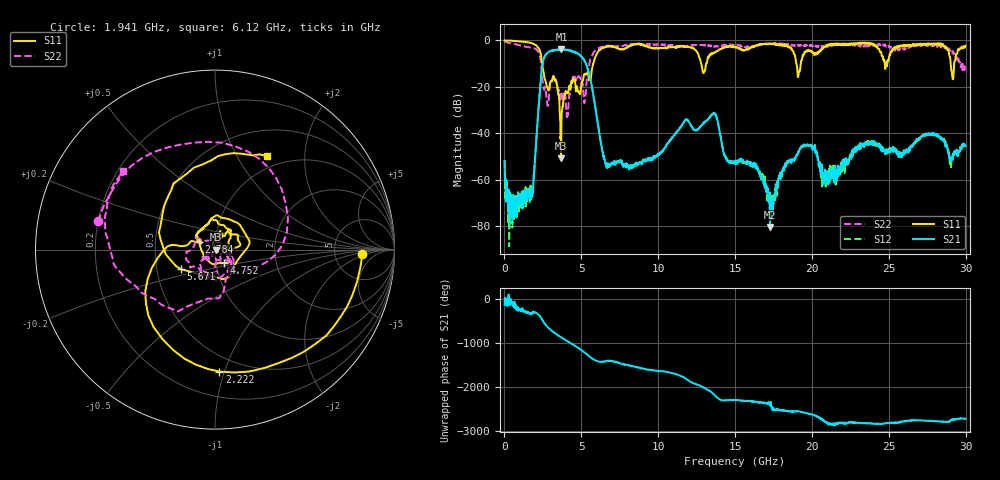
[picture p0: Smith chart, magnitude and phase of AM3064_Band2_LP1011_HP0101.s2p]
# Hz S DB R 50.0
!freq dBS11 angS11 dBS21 angS21 dBS12 angS12 dBS22 angS22
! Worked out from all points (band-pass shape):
!   1600 points, 10 MHz to 29.98 GHz, reference 50 ohm
!   highest |S21| = -3.77 dB at 3.703 GHz (marker M1); lowest = -80.2 dB at 17.27 GHz (marker M2)
!   |S21| within 3 dB of the highest: 2.628 GHz to 4.979 GHz (2.351 GHz wide, 61.8 % of centre)
!   lowest |S11| = -50.7 dB at 3.684 GHz (marker M3), VSWR 1.01, Z = 50.3 + j0.055 ohm
!   |S11| at or under -10 dB: 2.45 GHz to 5.773 GHz (3.323 GHz wide, 80.8 % of centre); 12.8 GHz to 13.12 GHz (321.1 MHz wide, 2.48 % of centre); 18.98 GHz to 19.27 GHz (290.4 MHz wide, 1.52 % of centre)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
!   |S22| runs from -33.0 to -0.3 dB; largest |S21 - S12| = 0.02
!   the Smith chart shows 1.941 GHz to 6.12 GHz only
!   S11 on the Smith chart (normalised r, x): 1.941 GHz: 10, -1; 2.222 GHz: 0.38, -0.96; 2.784 GHz: 0.83, +0.07; 4.752 GHz: 1.09, -0.16; 5.671 GHz: 0.67, -0.15; 6.12 GHz: 0.83, +1.34
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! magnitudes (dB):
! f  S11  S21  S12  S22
! 10 MHz  0.0  -51.8  -51.9  -0.3
! 647.3 MHz  -0.3  -72.9  -67.0  -1.5
! 1.941 GHz  -1.7  -55.8  -55.8  -3.5
! 2.222 GHz  -3.3  -28.8  -28.7  -5.0
! 2.784 GHz  -20.2  -5.4  -5.4  -27.7
! 3.29 GHz  -16.8  -4.2  -4.1  -17.2
! 3.684 GHz  -50.7  -4.0  -3.8  -23.5
! 3.703 GHz  -36.3  -3.8  -3.9  -23.0
! 4.752 GHz  -21.2  -5.6  -5.6  -15.8
! 5.015 GHz  -18.0  -7.1  -7.0  -18.6
! 5.671 GHz  -13.2  -19.4  -19.2  -7.2
! 6.12 GHz  -4.5  -37.8  -37.7  -3.4
! 6.702 GHz  -2.7  -54.8  -54.8  -2.5
! 10 GHz  -3.4  -48.5  -48.9  -1.9
! 13.6 GHz  -5.3  -31.6  -31.3  -2.6
! 15 GHz  -2.6  -52.7  -53.2  -1.9
! 17.27 GHz  -1.5  -80.2  -66.8  -1.3
! 19.99 GHz  -4.7  -46.1  -45.6  -1.9
! 20.82 GHz  -2.8  -59.6  -57.6  -2.3
! 25 GHz  -8.1  -48.3  -48.4  -2.3
! 29.18 GHz  -16.7  -50.3  -49.7  -4.9
! 29.98 GHz  -2.3  -45.5  -44.9  -10.4
